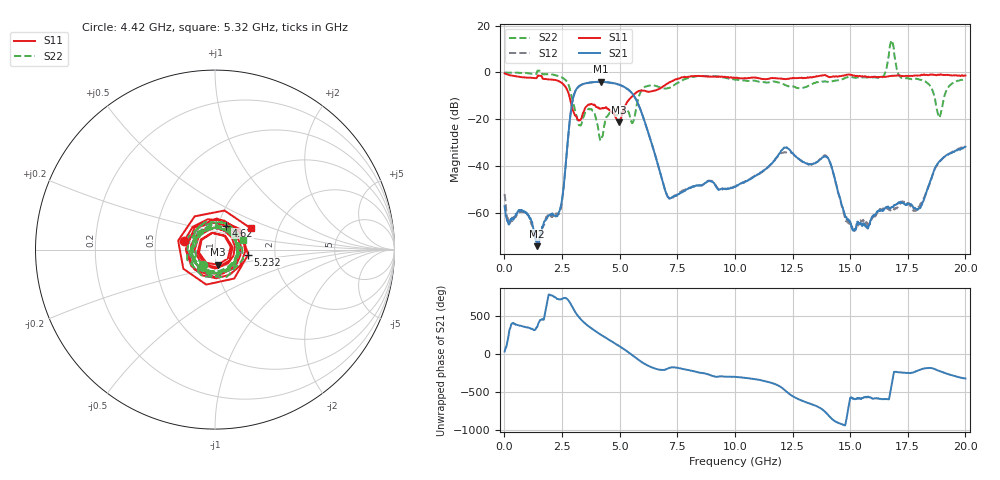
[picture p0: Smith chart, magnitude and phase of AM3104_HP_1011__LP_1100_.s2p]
!Created with skrf (http://scikit-rf.org).
# Hz S RI R 50.0
!freq ReS11 ImS11 ReS21 ImS21 ReS12 ImS12 ReS22 ImS22
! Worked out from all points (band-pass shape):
!   1601 points, 10 MHz to 20 GHz, reference 50 ohm
!   highest |S21| = -3.93 dB at 4.17 GHz (marker M1); lowest = -74.1 dB at 1.422 GHz (marker M2)
!   |S21| within 3 dB of the highest: 3.14 GHz to 5.324 GHz (2.184 GHz wide, 51.6 % of centre)
!   lowest |S11| = -21.3 dB at 4.958 GHz (marker M3), VSWR 1.19, Z = 50.9 - j8.68 ohm
!   |S11| at or under -10 dB: 2.818 GHz to 5.568 GHz (2.75 GHz wide, 65.6 % of centre)
!   |S22| runs from -29.0 to 13.6 dB; largest |S21 - S12| = 0.058
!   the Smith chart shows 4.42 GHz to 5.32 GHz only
!   S11 on the Smith chart (normalised r, x): 4.42 GHz: 0.70, +0.07; 4.62 GHz: 1.09, +0.30; 5.232 GHz: 1.45, -0.08; 5.32 GHz: 1.44, +0.36
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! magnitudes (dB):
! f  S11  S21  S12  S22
! 10 MHz  -0.4  -57.0  -51.8  0.0
! 1.422 GHz  -2.0  -74.1  -71.7  0.4
! 2.421 GHz  -4.0  -58.2  -59.2  -1.8
! 2.934 GHz  -14.8  -13.3  -13.4  -10.9
! 3.346 GHz  -19.5  -5.2  -5.3  -22.0
! 4.17 GHz  -15.5  -3.9  -4.0  -29.0
! 4.42 GHz  -14.9  -4.2  -4.2  -19.1
! 4.62 GHz  -16.6  -4.3  -4.4  -17.6
! 4.958 GHz  -21.3  -5.1  -5.2  -18.3
! 5.232 GHz  -14.6  -6.4  -6.4  -15.6
! 5.32 GHz  -12.7  -6.9  -6.9  -15.8
! 6.682 GHz  -7.2  -40.0  -40.1  -6.1
! 7.169 GHz  -4.1  -53.7  -53.9  -6.5
! 10.01 GHz  -2.4  -48.8  -48.7  -3.1
! 12.18 GHz  -2.8  -32.0  -34.1  -5.4
! 13.34 GHz  -2.1  -39.2  -39.2  -5.0
! 14.03 GHz  -1.7  -36.4  -36.3  -4.0
! 15.14 GHz  -1.2  -67.4  -67.2  -2.1
! 16.68 GHz  -1.6  -57.6  -58.4  7.3
! 18 GHz  -1.3  -57.9  -57.2  -3.0
! 18.86 GHz  -1.0  -38.1  -38.4  -19.3
! 20 GHz  -1.3  -31.7  -31.4  -2.8
